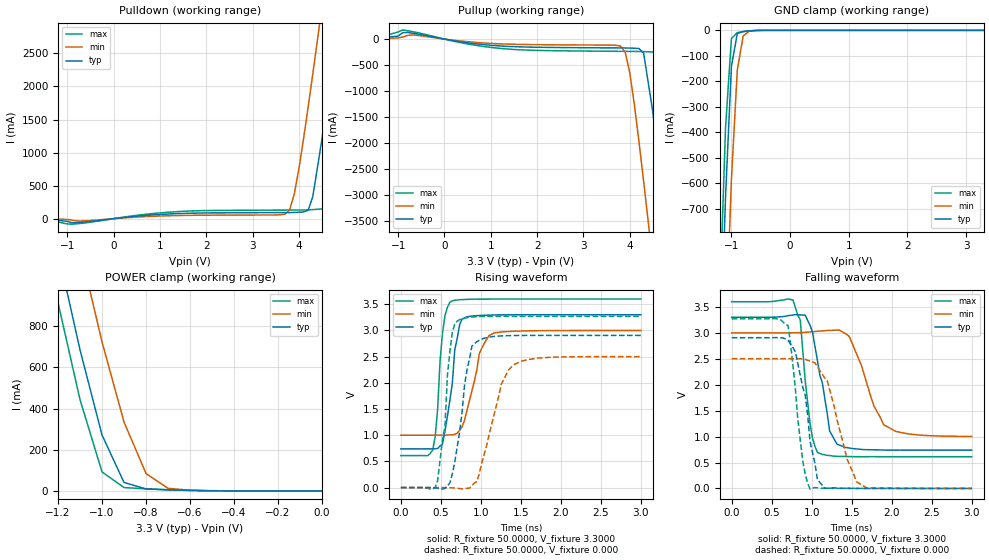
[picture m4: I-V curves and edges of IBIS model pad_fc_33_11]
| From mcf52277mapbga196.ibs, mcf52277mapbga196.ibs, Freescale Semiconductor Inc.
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|   Model Pad_fc_11
[Model]   pad_fc_33_11
Model_type   3-state
Polarity   Non-Inverting
Enable   Active-High
C_comp   5.5000pF   5.5000pF   5.5000pF
[Temperature Range]   25.0000   0.1500k   -40.0000
[Voltage Range]   3.3000V   3.0000V   3.6000V
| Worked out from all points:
|   slope of the pulldown table from 0 to 0.495 V, typ, clamps not added: 13.3 ohm
|   slope of the pullup table from 0 to 0.495 V, typ, clamps not added: 7.01 ohm
|   GND clamp passes 1 mA (typ) near -0.63 V on its own axis
|   POWER clamp passes 1 mA (typ) near -0.52 V on its own axis
|   rising waveform, R_fixture 50.0000, V_fixture 3.3000: 20-80 % time 126ps typ, 178ps min, 82.5ps max; typ from 0.738 V to 3.3 V
|   rising waveform, R_fixture 50.0000, V_fixture 0.000: 20-80 % time 154ps typ, 248ps min, 114ps max; typ from 0 V to 2.91 V
|   falling waveform, R_fixture 50.0000, V_fixture 3.3000: 20-80 % time 176ps typ, 286ps min, 113ps max; typ from 3.3 V to 0.738 V
|   falling waveform, R_fixture 50.0000, V_fixture 0.000: 20-80 % time 189ps typ, 253ps min, 131ps max; typ from 2.91 V to 0 V
[Pulldown]
| voltage   I(typ)   I(min)   I(max)
-3.3V     -2.5mA     -1.48mA    -3.04mA
-900mV    -62.09mA   -23.28mA   -83.07mA
3.7V      91.68mA    67.3mA     129.8mA
3.9V      94.19mA    373.4mA    130.3mA
4.2V      127mA      1.693A     133.4mA
4.3V      335.7mA    2.194A     137mA
4.5V      1.215A     3.217A     147.9mA
4.7V      2.235A     4.252A     525.6mA
4.9V      3.283A     5.291A     1.494A
5.1V      4.34A      6.331A     2.542A
5.3V      5.4A       7.372A     3.607A
6.6V      12.31A     14.15A     10.58A
[Pullup]
| voltage   I(typ)   I(min)   I(max)
-3.3V     5.7mA      5.8mA      5.8mA
-900mV    122.5mA    38.96mA    174.9mA
1.2V      -132.4mA   -91.65mA   -178.9mA
3.8V      -170.7mA   -134.8mA   -236mA
3.9V      -171.5mA   -247mA     -236.6mA
4V        -173.3mA   -645.5mA   -237.2mA
4.3V      -272.7mA   -2.742A    -240.9mA
4.5V      -1.418A    -4.31A     -248.5mA
4.7V      -2.976A    -5.903A    -508.1mA
4.9V      -4.597A    -7.5A      -1.92A
5.1V      -6.234A    -9.097A    -3.54A
6.6V      -18.53A    -21.08A    -16A
[GND_clamp]
| voltage   I(typ)   I(min)   I(max)
-3.3V     -18.48A    -18.65A    -18.42A
-1.2V     -1.357A    -1.942A    -1.067A
-1.1V     -650.5mA   -1.219A    -380mA
-1V       -141.2mA   -584.4mA   -32.29mA
-900mV    -12.85mA   -155.8mA   -8.89mA
-800mV    -4.42mA    -21.92mA   -5.229mA
-700mV    -2.049mA   -3.904mA   -2.397mA
-400mV    -7.776uA   -47.99uA   -2.574uA
3.3V      2.182uA    34.68uA    1.661uA
[POWER_clamp]
| voltage   I(typ)   I(min)   I(max)
-3.3V     12.25A     12.55A     12.11A
-1.3V     1.667A     2.163A     1.421A
-1.2V     1.163A     1.662A     913.9mA
-1.1V     684.8mA    1.177A     443.1mA
-1V       271.3mA    723.4mA    92.34mA
-900mV    41.22mA    334.1mA    16.32mA
-800mV    9.5mA      84.35mA    10.09mA
-700mV    5.131mA    12.62mA    5.713mA
-600mV    2.291mA    3.317mA    2.385mA
-500mV    581uA      1.097mA    477.4uA
0V        2.182uA    2.618uA    2.249uA
[Ramp]
| variable   typ   min   max
dV/dt_r   1.7436/0.1471n   1.5006/0.2462n   1.9622/0.1035n
dV/dt_f   1.5370/0.1701n   1.1982/0.2786n   1.7931/0.1222n
R_load = 50.0000
[Rising Waveform]
R_fixture = 50.0000
V_fixture = 3.3000
V_fixture_min = 3.0000
V_fixture_max = 3.6000
| time   V(typ)   V(min)   V(max)
0s        738.3mV    1.001V     611.5mV
398ps     739.4mV    1.001V     719.1mV
459.2ps   747.6mV    1.001V     1.493V
520.4ps   832.3mV    1.001V     2.952V
612.2ps   1.665V     1.006V     3.54V
673.5ps   2.629V     1.017V     3.578V
765.3ps   3.218V     1.162V     3.59V
979.6ps   3.286V     2.555V     3.599V
1.102ns   3.294V     2.904V     3.599V
3ns       3.3V       3V         3.6V
[Rising Waveform]
R_fixture = 50.0000
V_fixture = 0.000
| time   V(typ)   V(min)   V(max)
0s        770.8pV    311nV      29pV
459.2ps   -11.68mV   211.6uV    129.9mV
551ps     -14.01mV   484.7uV    1.169V
612.2ps   87.59mV    -2.831mV   2.596V
704.1ps   775.9mV    -12.97mV   3.178V
826.5ps   2.252V     -13.81mV   3.245V
949ps     2.784V     114mV      3.265V
1.255ns   2.896V     1.973V     3.27V
1.408ns   2.903V     2.345V     3.27V
3ns       2.906V     2.501V     3.27V
[Falling Waveform]
R_fixture = 50.0000
V_fixture = 3.3000
V_fixture_min = 3.0000
V_fixture_max = 3.6000
| time   V(typ)   V(min)   V(max)
0s        3.3V       3V         3.6V
765.3ps   3.343V     3.001V     3.633V
857.1ps   3.346V     3.004V     3.247V
979.6ps   3.143V     3.017V     1.243V
1.071ns   2.462V     3.03V      695.1mV
1.225ns   1.107V     3.047V     634mV
1.316ns   854.2mV    3.051V     619.3mV
1.469ns   779.5mV    2.929V     614.5mV
1.898ns   740.8mV    1.229V     611.6mV
3ns       738.3mV    1.003V     611.5mV
[Falling Waveform]
R_fixture = 50.0000
V_fixture = 0.000
| time   V(typ)   V(min)   V(max)
0s        2.906V     2.502V     3.271V
704.1ps   2.855V     2.502V     3.139V
795.9ps   2.634V     2.501V     1.917V
887.8ps   1.951V     2.496V     535.1mV
918.4ps   1.802V     2.487V     277.5mV
979.6ps   904.9mV    2.456V     -13.71mV
1.071ns   170.2mV    2.346V     10.69mV
1.163ns   1.501mV    2.128V     5.184mV
1.561ns   1.889mV    127.8mV    95.73uV
3ns       509.2nV    97.31uV    -326.6nV
